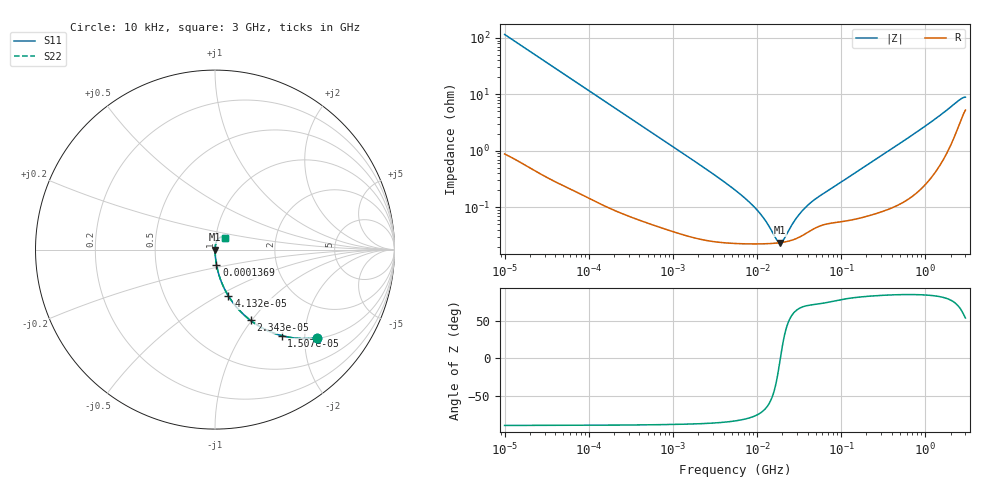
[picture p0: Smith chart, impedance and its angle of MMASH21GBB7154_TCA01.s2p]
! MMASH21GBB7154_TCA01  S-PARAMETER MODEL  ( Standard Model )
! Model Generated by TAIYO YUDEN Corporation (http://www.ty-top.com)
! Version 1.0
! TAIYO YUDEN Control No. 220601
! Copyright(c) 2019 TAIYO YUDEN CO.,LTD. All Rights Reserved.
! Product Description (link to TY-COMPAS)
! https://ds.yuden.co.jp/TYCOMPAS/or/detail?pn=MMASH21GBB7154KTCA01&u=M
! Products Name : Multilayer Ceramic Capacitors
! Characteristics :
!  Capacitance : 0.15 [uF] , Rated Voltage : 100 [V] , TCC : X7R
!  Case Size : 2.0 x 1.25 / 0.079 x 0.049 [mm/inch] , Thickness : 1.25 / 0.049 [mm/inch]
!  (Conditions: Temperature = 25 [degC] , DC Bias Voltage = 0 [V])
! External Node Assignments :
!  1  o---| |---o  2
! GND o---------o GND
! Frequency Range : 10kHz  -  3GHz  [ 401 STEP ]
# MHZ S RI R 50
! Freq[MHz].  S11 Real  S11 Imag  S21 Real  S21 Imag  S12 Real  S12 Imag  S22 Real  S22 Imag
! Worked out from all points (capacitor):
!   401 points, 10 kHz to 3 GHz, reference 50 ohm
!   read as one part in series: C = 138 nF near 10.65 kHz
!   lowest |Z| = 23.6 mohm at 18.73 MHz (marker M1)
!   series resonance near 18.95 MHz, so ESL is about 510 pH
!   S11 on the Smith chart (normalised r, x): 10 kHz: 1.02, -2.30; 15.07 kHz: 1.01, -1.53; 23.43 kHz: 1.01, -0.99; 41.32 kHz: 1.01, -0.56; 136.9 kHz: 1.00, -0.17; 3 GHz: 1.11, +0.14
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0.01  0.5693 -0.4914  0.4307 0.4914  0.4307 0.4914  0.5693 -0.4914
0.015066  0.3706 -0.4788  0.6294 0.4788  0.6294 0.4788  0.3706 -0.4788
0.023426  0.198 -0.3941  0.802 0.3941  0.802 0.3941  0.198 -0.3941
0.041322  0.0752 -0.2588  0.9248 0.2588  0.9248 0.2588  0.0752 -0.2588
0.082683  0.021 -0.1377  0.979 0.1377  0.979 0.1377  0.021 -0.1377
0.136931  0.00836 -0.0845  0.9916 0.0845  0.9916 0.0845  0.00836 -0.0845
0.683653  0.000745 -0.0173  0.9993 0.0173  0.9993 0.0173  0.000745 -0.0173
2.652321  0.000274 -0.00443  0.9997 0.00443  0.9997 0.00443  0.000274 -0.00443
5.477226  0.000233 -0.00201  0.9998 0.00201  0.9998 0.00201  0.000233 -0.00201
7.747855  0.000227 -0.00129  0.9998 0.00129  0.9998 0.00129  0.000227 -0.00129
10.29003  0.000225 -0.000827  0.9998 0.000827  0.9998 0.000827  0.000225 -0.000827
12.83117  0.000226 -0.00051  0.9998 0.00051  0.9998 0.00051  0.000226 -0.00051
17.04125  0.000232 -0.000136  0.9998 0.000136  0.9998 0.000136  0.000232 -0.000136
18.73182  0.000236 -1.49e-05  0.9998 1.49e-05  0.9998 1.49e-05  0.000236 -1.49e-05
20.5901  0.000241 0.000106  0.9998 -0.000106  0.9998 -0.000106  0.000241 0.000106
26.49725  0.000264 0.000438  0.9997 -0.000438  0.9997 -0.000438  0.000264 0.000438
32.0153  0.000297 0.0007  0.9997 -0.0007  0.9997 -0.0007  0.000297 0.0007
45.28751  0.000402 0.0012  0.9996 -0.0012  0.9996 -0.0012  0.000402 0.0012
374.4521  0.00104 0.0101  0.999 -0.0101  0.999 -0.0101  0.00104 0.0101
1128.871  0.00404 0.0308  0.996 -0.0308  0.996 -0.0308  0.00404 0.0308
2482.93  0.031 0.0685  0.969 -0.0685  0.969 -0.0685  0.031 0.0685
3000  0.0544 0.0649  0.9456 -0.0649  0.9456 -0.0649  0.0544 0.0649
